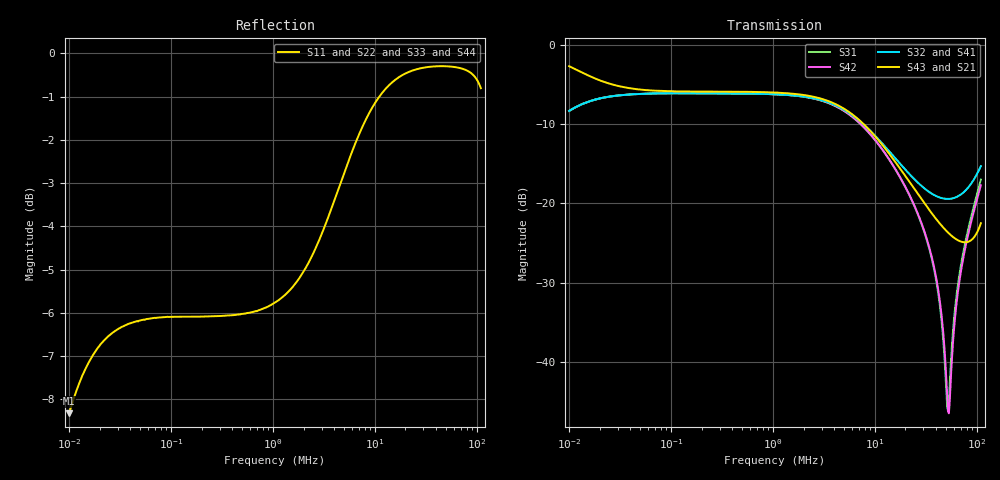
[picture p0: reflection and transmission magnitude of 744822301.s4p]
! Touchstone file was created by TriD Version 2018.1.1 (64-bit) (04.05.2018)
! (C) EMCoS 1999-2018
! Project : TRID_WE_CMB_S_744_822_301_Task 1\Task 1.in
! Date  : 2018-06-18  22:07:17
# HZ S RI R  50.00
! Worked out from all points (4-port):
!   503 points, 10 kHz to 110 MHz, reference 50 ohm
!   strongest paths, dB at 10 kHz, 101.6 kHz, 1.05 MHz, 10.85 MHz, 110 MHz:
!     S43: -2.7, -5.9, -6.0, -12.0, -22.5
!     S21: -2.7, -5.9, -6.0, -12.0, -22.5
!     S32: -8.4, -6.1, -6.3, -11.9, -15.3
!     S41: -8.4, -6.1, -6.3, -11.9, -15.3
!     S42: -8.4, -6.1, -6.3, -12.5, -17.7
!     S31: -8.4, -6.1, -6.3, -12.6, -17.0
!   lowest |S11| = -8.3 dB at 10 kHz (marker M1), VSWR 2.24, Z = 79.6 + j43.2 ohm
!   |S11| at or under -10 dB: nowhere
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10000  0.3058 0.2314  0.6942 -0.2314  0.3056 0.2298  -0.3056 -0.2297
       0.6942 -0.2314  0.3058 0.2314  -0.3056 -0.2297  0.3056 0.2298
       0.3057 0.2297  -0.3057 -0.2297  0.3057 0.2314  0.6943 -0.2314
       -0.3057 -0.2297  0.3057 0.2297  0.6943 -0.2314  0.3057 0.2314
5883300  0.7285 0.2353  0.2714 -0.2478  0.2562 -0.2457  -0.256 0.2569
         0.2714 -0.2478  0.7285 0.2353  -0.256 0.2569  0.2562 -0.2458
         0.2562 -0.2458  -0.2561 0.2569  0.7285 0.2353  0.2714 -0.2478
         -0.2561 0.2569  0.2563 -0.2459  0.2714 -0.2478  0.7284 0.2353
3.062e7  0.9623 0.0278  0.0335 -0.0946  0.0121 -0.0647  -0.00796 0.1241
         0.0335 -0.0946  0.9623 0.0286  -0.00796 0.1241  0.0121 -0.0657
         0.0121 -0.0647  -0.00796 0.1241  0.9623 0.0278  0.0336 -0.0946
         -0.00796 0.1241  0.0121 -0.0657  0.0336 -0.0946  0.9623 0.0286
4.2745e7  0.9659 -0.0241  0.0254 -0.0711  0.00528 -0.0242  0.00331 0.1091
          0.0254 -0.0711  0.966 -0.0227  0.00331 0.1091  0.0052 -0.0257
          0.00528 -0.0242  0.00331 0.1091  0.9659 -0.0241  0.0254 -0.0712
          0.00331 0.1091  0.0052 -0.0257  0.0254 -0.0712  0.966 -0.0227
5.2411e7  0.9641 -0.0578  0.0219 -0.0616  0.00488 0.000497  0.00904 0.1062
          0.0219 -0.0616  0.9644 -0.0559  0.00904 0.1062  0.00461 -0.00156
          0.00488 0.000493  0.00904 0.1062  0.964 -0.0578  0.0219 -0.0616
          0.00904 0.1062  0.00461 -0.00156  0.0219 -0.0616  0.9644 -0.0559
6.6691e7  0.9567 -0.1029  0.017 -0.0556  0.00896 0.0322  0.0171 0.1101
          0.017 -0.0556  0.9577 -0.0999  0.0171 0.1101  0.00816 0.0291
          0.00896 0.0322  0.0171 0.1101  0.9567 -0.1029  0.017 -0.0556
          0.0171 0.1101  0.00816 0.0291  0.017 -0.0556  0.9577 -0.0999
1.1e8  0.8809 -0.2334  -0.0335 -0.0671  0.073 0.121  0.0784 0.1524
       -0.0335 -0.0671  0.8908 -0.2255  0.0784 0.1524  0.0643 0.1129
       0.073 0.121  0.0784 0.1524  0.8808 -0.2335  -0.0335 -0.0671
       0.0784 0.1524  0.0643 0.1129  -0.0335 -0.0671  0.8909 -0.2255
